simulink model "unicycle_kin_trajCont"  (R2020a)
settings: Solver=FixedStepAuto  StartTime=0.0  StopTime=inf  RelTol=1e-3
undefined symbols (not defined in the file or in its folder): Angular, cmd_vel, desired_position, desired_velocity, geometry_msgs, Linear, nav_msgs, odom, Odometry, Point, Twist
libraries: robotlib x5

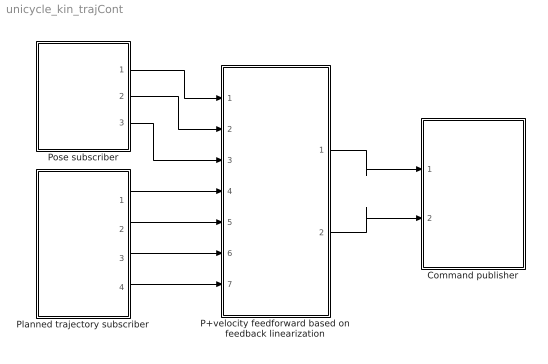
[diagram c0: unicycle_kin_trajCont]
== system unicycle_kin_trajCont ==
  Command publisher : Subsystem  mask{simPublishRate=25}
      mask prompts: simPublishRate "Publising rate [Hz]"
  P+velocity feedforward based on feedback linearization : Subsystem  mask{KP=1.5, P_dist=0.1}
      mask prompts: KP "Proportional gain"; P_dist "Point P distance"
  Planned trajectory subscriber : Subsystem
  Pose subscriber : Subsystem
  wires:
  P+velocity feedforward based on feedback linearization/1(v) -> Command publisher/1(v)
  P+velocity feedforward based on feedback linearization/2(w) -> Command publisher/2(w)
  Pose subscriber/1(x) -> P+velocity feedforward based on feedback linearization/1(x)
  Pose subscriber/2(y) -> P+velocity feedforward based on feedback linearization/2(y)
  Pose subscriber/3(theta) -> P+velocity feedforward based on feedback linearization/3(theta)
  Planned trajectory subscriber/4(dy) -> P+velocity feedforward based on feedback linearization/7(dyd)
  Planned trajectory subscriber/3(dx) -> P+velocity feedforward based on feedback linearization/6(dxd)
  Planned trajectory subscriber/1(x) -> P+velocity feedforward based on feedback linearization/4(xd)
  Planned trajectory subscriber/2(y) -> P+velocity feedforward based on feedback linearization/5(yd)

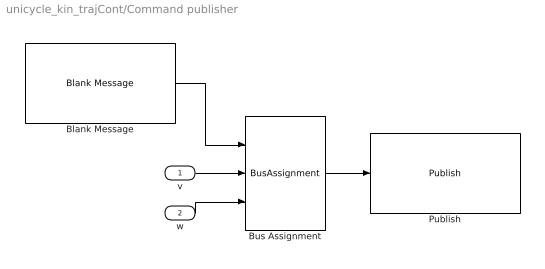
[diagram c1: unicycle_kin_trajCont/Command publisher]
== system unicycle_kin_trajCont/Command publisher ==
  v : Inport  SampleTime=1/simPublishRate
  w : Inport  Port=2  SampleTime=1/simPublishRate
  Blank Message : robotlib/Blank Message  messageClass=Message  entityType=geometry_msgs/Twist  messageType=geometry_msgs/Twist  SampleTime=1/simPublishRate
  Bus Assignment : BusAssignment  AssignedSignals=Linear.X,Angular.Z
  Publish : robotlib/Publish  topicSource=Specify your own  topic=/cmd_vel  messageType=geometry_msgs/Twist  messageQueueLength=1
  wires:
  Bus Assignment/1 -> Publish/1
  Blank Message/1 -> Bus Assignment/1
  v/1 -> Bus Assignment/2
  w/1 -> Bus Assignment/3

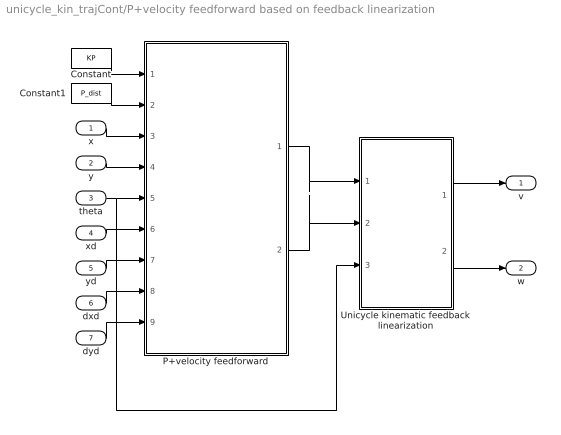
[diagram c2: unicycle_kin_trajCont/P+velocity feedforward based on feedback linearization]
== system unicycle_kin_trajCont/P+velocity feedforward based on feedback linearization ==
  x : Inport
  y : Inport  Port=2
  theta : Inport  Port=3
  xd : Inport  Port=4
  yd : Inport  Port=5
  dxd : Inport  Port=6
  dyd : Inport  Port=7
  Constant : Constant  Value=KP
  Constant1 : Constant  Value=P_dist
  P+velocity feedforward : MATLAB Function  TreatAsAtomicUnit=on
  Unicycle kinematic feedback linearization : Subsystem  mask{epsilon=0.1}
  v : Outport  VectorParamsAs1DForOutWhenUnconnected=off
  w : Outport  Port=2  VectorParamsAs1DForOutWhenUnconnected=off
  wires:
  dyd/1 -> P+velocity feedforward/9(dyd)
  Constant/1 -> P+velocity feedforward/1(KP)
  x/1 -> P+velocity feedforward/3(x)
  y/1 -> P+velocity feedforward/4(y)
  xd/1 -> P+velocity feedforward/6(xd)
  yd/1 -> P+velocity feedforward/7(yd)
  dxd/1 -> P+velocity feedforward/8(dxd)
  P+velocity feedforward/2(v_yP) -> Unicycle kinematic feedback linearization/2(v_yP)
  P+velocity feedforward/1(v_xP) -> Unicycle kinematic feedback linearization/1(v_xP)
  Unicycle kinematic feedback linearization/2(omega) -> w/1
  Unicycle kinematic feedback linearization/1(v) -> v/1
  theta/1 -> Unicycle kinematic feedback linearization/3(theta), P+velocity feedforward/5(theta)
  Constant1/1 -> P+velocity feedforward/2(P_dist)

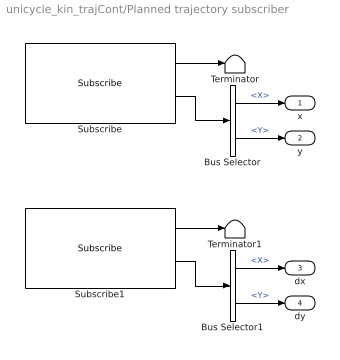
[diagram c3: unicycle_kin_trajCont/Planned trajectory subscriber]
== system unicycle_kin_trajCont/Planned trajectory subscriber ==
  Bus Selector : BusSelector  OutputSignals=X,Y
  Bus Selector1 : BusSelector  OutputSignals=X,Y
  Subscribe : robotlib/Subscribe  topicSource=Specify your own  topic=/desired_position  messageType=geometry_msgs/Point  sampleTime=-1  messageQueueLength=1
  Subscribe1 : robotlib/Subscribe  topicSource=Specify your own  topic=/desired_velocity  messageType=geometry_msgs/Point  sampleTime=-1  messageQueueLength=1
  Terminator : Terminator
  Terminator1 : Terminator
  x : Outport
  y : Outport  Port=2
  dx : Outport  Port=3
  dy : Outport  Port=4
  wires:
  Bus Selector/2 -> y/1  "<Y>"
  Subscribe/1 -> Terminator/1
  Subscribe/2 -> Bus Selector/1
  Bus Selector/1 -> x/1  "<X>"
  Bus Selector1/2 -> dy/1  "<Y>"
  Bus Selector1/1 -> dx/1  "<X>"
  Subscribe1/1 -> Terminator1/1
  Subscribe1/2 -> Bus Selector1/1

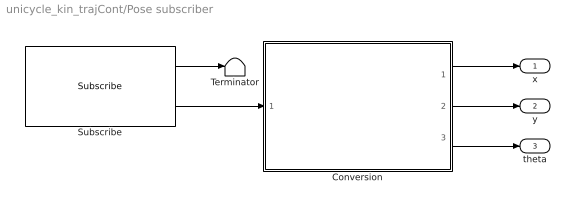
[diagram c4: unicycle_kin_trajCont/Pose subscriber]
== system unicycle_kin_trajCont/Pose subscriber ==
  Conversion : MATLAB Function  TreatAsAtomicUnit=on
  Subscribe : robotlib/Subscribe  topicSource=Specify your own  topic=/odom  messageType=nav_msgs/Odometry  sampleTime=-1  messageQueueLength=1
  Terminator : Terminator
  x : Outport
  y : Outport  Port=2
  theta : Outport  Port=3
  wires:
  Subscribe/1 -> Terminator/1
  Subscribe/2 -> Conversion/1(odomMsg)
  Conversion/1(x) -> x/1
  Conversion/2(y) -> y/1
  Conversion/3(theta) -> theta/1

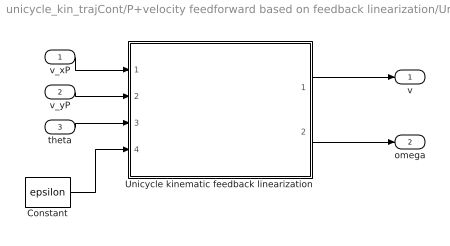
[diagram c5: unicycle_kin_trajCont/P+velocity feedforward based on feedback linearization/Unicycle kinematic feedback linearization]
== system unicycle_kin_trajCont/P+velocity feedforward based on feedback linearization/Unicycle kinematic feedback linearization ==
  v_xP : Inport
  v_yP : Inport  Port=2
  theta : Inport  Port=3
  Constant : Constant  Value=epsilon
  Unicycle kinematic feedback linearization : MATLAB Function  TreatAsAtomicUnit=on
  v : Outport  VectorParamsAs1DForOutWhenUnconnected=off
  omega : Outport  Port=2  VectorParamsAs1DForOutWhenUnconnected=off
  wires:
  Unicycle kinematic feedback linearization/2(w) -> omega/1
  v_yP/1 -> Unicycle kinematic feedback linearization/2(v_yP)
  Unicycle kinematic feedback linearization/1(v) -> v/1
  v_xP/1 -> Unicycle kinematic feedback linearization/1(v_xP)
  theta/1 -> Unicycle kinematic feedback linearization/3(theta)
  Constant/1 -> Unicycle kinematic feedback linearization/4(epsilon)

== matlab function unicycle_kin_trajCont/P+velocity feedforward
based on feedback linearization/Unicycle kinematic
feedback linearization/Unicycle kinematic feedback linearization ==
function [v,w] = fblin_unicycle_kinematic(v_xP,v_yP,theta,epsilon)

v = v_xP*cos(theta)+v_yP*sin(theta);
w = (v_yP*cos(theta)-v_xP*sin(theta))/epsilon;

== matlab function unicycle_kin_trajCont/P+velocity feedforward
based on feedback linearization/P+velocity feedforward ==
function [v_xP,v_yP] = P_velFeedforward(KP,P_dist,x,y,theta,xd,yd,dxd,dyd)

% Point P transformation
xP = x+P_dist*cos(theta);
yP = y+P_dist*sin(theta);

xPd = xd+P_dist*cos(theta);
yPd = yd+P_dist*sin(theta);

% Control law
v_xP = dxd + KP*(xPd-xP);
v_yP = dyd + KP*(yPd-yP);

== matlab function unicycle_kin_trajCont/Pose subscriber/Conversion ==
function [x,y,theta]  = odom_2_xytheta(odomMsg)

% Position
x = odomMsg.Pose.Pose.Position.X;
y = odomMsg.Pose.Pose.Position.Y;

% Orientation
orientation = [odomMsg.Pose.Pose.Orientation.X,odomMsg.Pose.Pose.Orientation.Y,...
    odomMsg.Pose.Pose.Orientation.Z,odomMsg.Pose.Pose.Orientation.W];

if all(orientation==zeros(1,4))
    theta = 0;
else
    eul = quat2eul(orientation,'ZYX');
    theta = eul(3);
end
